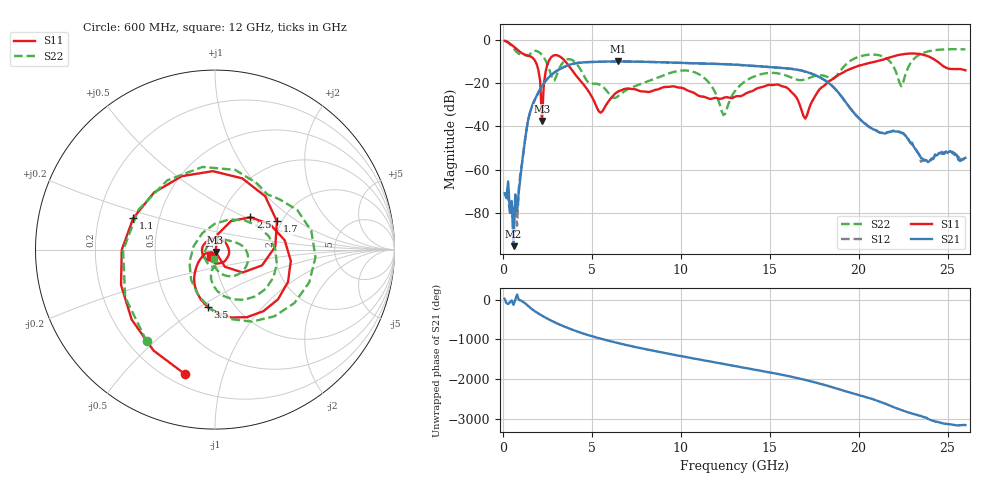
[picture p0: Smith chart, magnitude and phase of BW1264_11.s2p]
!Keysight Technologies,N5245B,MY57181159,A.13.60.06
!Date: Friday, December 18, 2020 23:52:29
!Correction: S11(Full 2 Port(1,2))
!S21(Full 2 Port(1,2))
!S12(Full 2 Port(1,2))
!S22(Full 2 Port(1,2))
!S2P File: Measurements: S11, S21, S12, S22:
# Hz S  dB  R 50
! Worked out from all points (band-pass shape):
!   260 points, 100 MHz to 26 GHz, reference 50 ohm
!   highest |S21| = -9.93 dB at 6.5 GHz (marker M1); lowest = -95.5 dB at 600 MHz (marker M2)
!   |S21| within 3 dB of the highest: 3.329 GHz to 15.7 GHz (12.37 GHz wide, 130 % of centre)
!   lowest |S11| = -37.5 dB at 2.2 GHz (marker M3), VSWR 1.03, Z = 50.3 - j1.3 ohm
!   |S11| at or under -10 dB: 1.832 GHz to 2.572 GHz (739.9 MHz wide, 33.6 % of centre); 3.52 GHz to 20.95 GHz (17.43 GHz wide, 142 % of centre); 24.43 GHz to end of sweep
!   |S22| runs from -34.8 to -0.2 dB; largest |S21 - S12| = 0.0006
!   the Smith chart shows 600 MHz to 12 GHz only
!   S11 on the Smith chart (normalised r, x): 600 MHz: 0.27, -0.75; 1.1 GHz: 0.35, +0.16; 1.7 GHz: 1.88, +0.70; 2.5 GHz: 1.37, +0.53; 3.5 GHz: 0.76, -0.54; 12 GHz: 0.94, -0.07
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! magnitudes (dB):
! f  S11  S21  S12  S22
! 100 MHz  -0.4  -71.1  -70.8  -0.2
! 300 MHz  -1.1  -65.5  -74.0  -1.2
! 600 MHz  -2.9  -95.5  -79.0  -3.9
! 800 MHz  -4.3  -79.3  -86.1  -5.8
! 1.1 GHz  -6.2  -55.6  -56.4  -6.6
! 1.7 GHz  -8.4  -29.5  -29.5  -5.2
! 2.1 GHz  -19.1  -22.8  -22.7  -6.1
! 2.2 GHz  -37.5  -21.4  -21.4  -6.9
! 2.5 GHz  -11.5  -18.0  -18.0  -11.2
! 3.5 GHz  -9.8  -12.3  -12.3  -9.5
! 4.5 GHz  -20.2  -10.4  -10.4  -15.7
! 5.5 GHz  -33.7  -10.0  -10.0  -20.9
! 6.5 GHz  -23.8  -9.9  -9.9  -25.9
! 8.8 GHz  -22.6  -10.3  -10.3  -17.1
! 12 GHz  -26.8  -11.0  -11.0  -25.5
! 12.4 GHz  -26.8  -11.2  -11.2  -34.8
! 13.1 GHz  -26.1  -11.4  -11.4  -23.1
! 17.4 GHz  -28.2  -15.7  -15.7  -17.0
! 21.7 GHz  -8.2  -42.7  -42.5  -9.4
! 22.4 GHz  -6.7  -43.0  -42.9  -21.4
! 23.4 GHz  -6.4  -53.2  -53.0  -6.9
! 26 GHz  -14.0  -54.6  -55.5  -4.3
